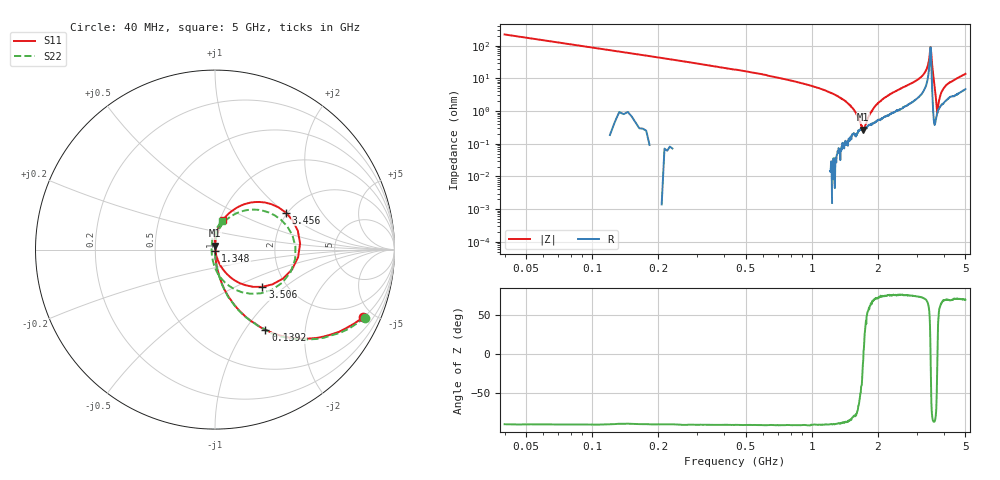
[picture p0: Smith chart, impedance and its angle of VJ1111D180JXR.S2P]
! VJ1111D180JXR
! DATE 02/16/2022  10:11
! CAPACITORS MOUNTED IN SERIES ON 25 MIL THICK MICROSTRIP SUBSTRATE
# GHz  S  MA  R  50.00
!  FREQ  S11M  S11A  S21M  S21A  S12M  S12A  S22M  S22A
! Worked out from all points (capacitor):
!   801 points, 40 MHz to 5 GHz, reference 50 ohm
!   read as one part in series: C = 18 pF near 64.8 MHz
!   lowest |Z| = 268 mohm at 1.708 GHz (marker M1)
!   series resonance near 1.718 GHz, so ESL is about 480 pH
!   S11 on the Smith chart (normalised r, x): 40 MHz: 1.02, -4.38; 139.2 MHz: 1.00, -1.25; 1.348 GHz: 1.00, -0.02; 3.456 GHz: 1.96, +1.01; 3.506 GHz: 1.52, -0.71; 5 GHz: 1.04, +0.35
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0.04  0.9081 -24.5  0.415 65.3  0.4144 65.4  0.916 -24.4
0.1392  0.5287 -57.9  0.8428 31.8  0.8531 33.6  0.5331 -57.3
0.3314  0.2438 -75.7  0.9692 14.6  0.9748 14.4  0.2463 -75.8
0.8708  0.06399 -85.2  0.9979 5.0  1.002 4.9  0.06421 -86.1
1.1684  0.02652 -85.0  0.9972 3.3  1.002 3.1  0.02629 -87.8
1.3482  0.007912 -79.4  0.9974 2.5  1.002 2.3  0.00848 -88.5
1.4474  0.001125 -3.2  0.9952 2.2  1.001 1.9  0.0002868 -176.1
1.4908  0.004036 74.7  0.9956 2.0  1 1.9  0.00406 80.8
1.5342  0.007606 78.2  0.9953 1.9  0.9992 1.7  0.007242 88.0
1.6954  0.02024 85.7  0.9939 1.4  0.9984 1.2  0.01999 87.5
1.7078  0.02111 85.9  0.9935 1.4  0.9989 1.2  0.02102 87.7
2.52  0.07602 83.9  0.9786 -0.7  0.9846 -0.9  0.07581 84.3
3.3508  0.2252 67.8  0.8925 -7.9  0.8962 -7.9  0.2152 62.8
3.4562  0.4452 27.6  0.5812 -9.1  0.5841 -9.2  0.4226 18.0
3.5058  0.3358 -38.2  0.7981 22.4  0.8028 22.3  0.3158 -51.2
3.574  0.07597 -73.1  0.9734 9.3  0.9783 9.1  0.07574 -96.6
3.6174  0.01641 -76.3  0.9803 6.0  0.9852 5.9  0.02847 -129.7
3.6422  0.003757 73.3  0.9795 4.8  0.9856 4.7  0.01916 -173.2
3.698  0.03476 92.5  0.9752 3.1  0.9803 3.0  0.031 124.5
3.7724  0.06364 90.8  0.9673 2.0  0.9715 2.0  0.05278 108.3
4.1754  0.1145 80.0  0.9589 -1.0  0.964 -1.1  0.09897 83.8
5  0.1712 74.3  0.9256 -4.2  0.931 -4.3  0.1612 76.3
